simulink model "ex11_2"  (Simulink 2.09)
settings: Solver=ode5  StartTime=0.0  StopTime=100  FixedStep=0.1  RelTol=1e-3  AbsTol=1e-6

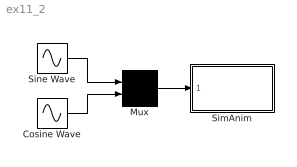
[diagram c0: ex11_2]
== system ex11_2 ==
  Cosine Wave : Sin  Amplitude=1  Frequency=1  Phase=pi/2  SampleTime=0
  Mux : Mux  Inputs=2
  SimAnim : Subsystem
  Sine Wave : Sin  Amplitude=1  Frequency=1  Phase=0  SampleTime=0
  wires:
  Mux/1 -> SimAnim/1(in_1)
  Sine Wave/1 -> Mux/1
  Cosine Wave/1 -> Mux/2

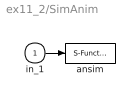
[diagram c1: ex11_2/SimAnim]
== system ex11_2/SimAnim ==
  in_1 : Inport  Port=1  PortWidth=-1  SampleTime=-1
  ansim : S-Function  FunctionName=ansim  Parameters=1
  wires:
  in_1/1 -> ansim/1
